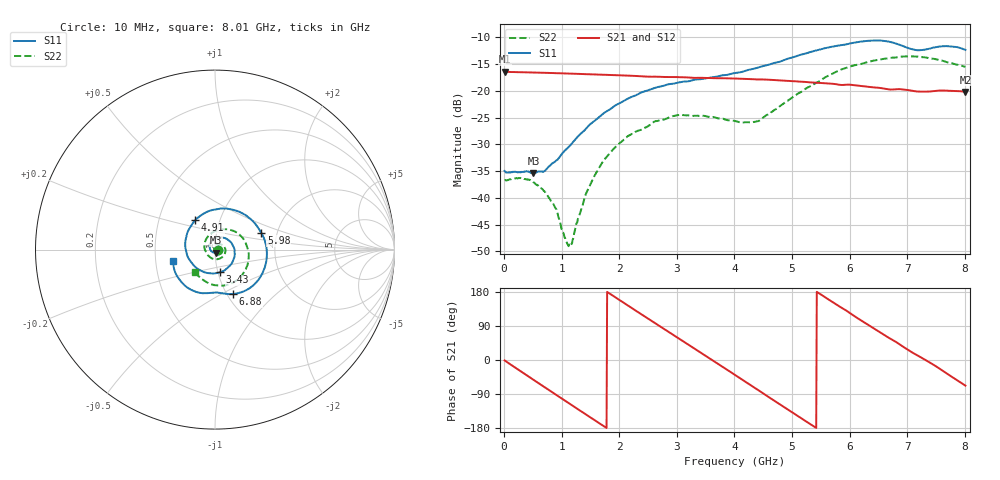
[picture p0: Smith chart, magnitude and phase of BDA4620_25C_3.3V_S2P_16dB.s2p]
!Agilent Technologies,E5071B,MY42404982,A.09.10
!Date: Wed May 06 08:52:02 2026
!Data & Calibration Information:
!Freq	S11:SOLT2(ON)	S21:SOLT2(ON)	S12:SOLT2(ON)	S22:SOLT2(ON)
# Hz S RI R 50
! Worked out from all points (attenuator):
!   801 points, 10 MHz to 8.01 GHz, reference 50 ohm
!   highest |S21| = -16.42 dB at 10 MHz (marker M1); lowest = -20.2 dB at 8.01 GHz (marker M2)
!   lowest |S11| = -35.4 dB at 510 MHz (marker M3), VSWR 1.03, Z = 50.3 - j1.68 ohm
!   |S11| at or under -10 dB: start of sweep to end of sweep
!   |S22| runs from -49.0 to -13.6 dB; largest |S21 - S12| = 0.00069
!   S11 on the Smith chart (normalised r, x): 10 MHz: 1.04, -0.00; 3.43 GHz: 1.03, -0.26; 4.91 GHz: 0.76, +0.26; 5.98 GHz: 1.66, +0.33; 6.88 GHz: 1.07, -0.57; 8.01 GHz: 0.62, -0.08
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1e7  0.0178 -0.00132  0.151 -0.00322  0.1512 -0.00322  0.0146 -0.000529
5.1e8  0.00331 -0.0166  0.0911 -0.1169  0.0912 -0.1171  0.0124 -0.00655
8.7e8  -0.0186 -0.0109  0.00403 -0.1463  0.00401 -0.1466  0.00335 -0.00775
1.12e9  -0.0291 0.00657  -0.0578 -0.133  -0.0581 -0.1331  -0.00274 -0.00223
1.18e9  -0.0299 0.0123  -0.0713 -0.1258  -0.0716 -0.126  -0.00373 -0.000288
1.35e9  -0.0289 0.0285  -0.1044 -0.0988  -0.1045 -0.0988  -0.00569 0.00575
1.58e9  -0.0165 0.0502  -0.1332 -0.0498  -0.1334 -0.0498  -0.00462 0.0157
1.87e9  0.0153 0.0672  -0.1388 0.0204  -0.1392 0.0205  0.00419 0.0271
2.16e9  0.0562 0.0638  -0.1104 0.0838  -0.1106 0.0838  0.0199 0.0323
2.68e9  0.1088 -0.00177  -0.00443 0.1352  -0.00429 0.1354  0.0489 0.0189
3.43e9  0.0294 -0.1255  0.1257 0.0411  0.1259 0.041  0.0431 -0.0393
4.01e9  -0.1103 -0.0964  0.1005 -0.0827  0.1007 -0.0829  -0.0157 -0.0499
4.41e9  -0.1648 0.00985  0.0241 -0.1253  0.0241 -0.1257  -0.0504 -0.013
4.91e9  -0.11 0.1647  -0.0781 -0.0963  -0.0782 -0.0966  -0.0441 0.0668
5.35e9  0.0428 0.2291  -0.1186 -0.0159  -0.1187 -0.0159  0.0251 0.1097
5.98e9  0.2582 0.0922  -0.0676 0.0921  -0.0677 0.0921  0.1528 0.0668
6.33e9  0.2846 -0.0706  -0.00321 0.1089  -0.00312 0.109  0.1862 -0.0102
6.68e9  0.1888 -0.2176  0.0537 0.0879  0.0539 0.0881  0.1753 -0.1001
6.88e9  0.1019 -0.2475  0.0794 0.0666  0.0795 0.0669  0.1485 -0.1457
7.19e9  0.00646 -0.239  0.0967 0.0187  0.0969 0.0188  0.0746 -0.1948
7.54e9  -0.1087 -0.2343  0.0939 -0.0355  0.0941 -0.0353  -0.0184 -0.1935
8.01e9  -0.2323 -0.0643  0.0372 -0.0904  0.0374 -0.0905  -0.1126 -0.123
